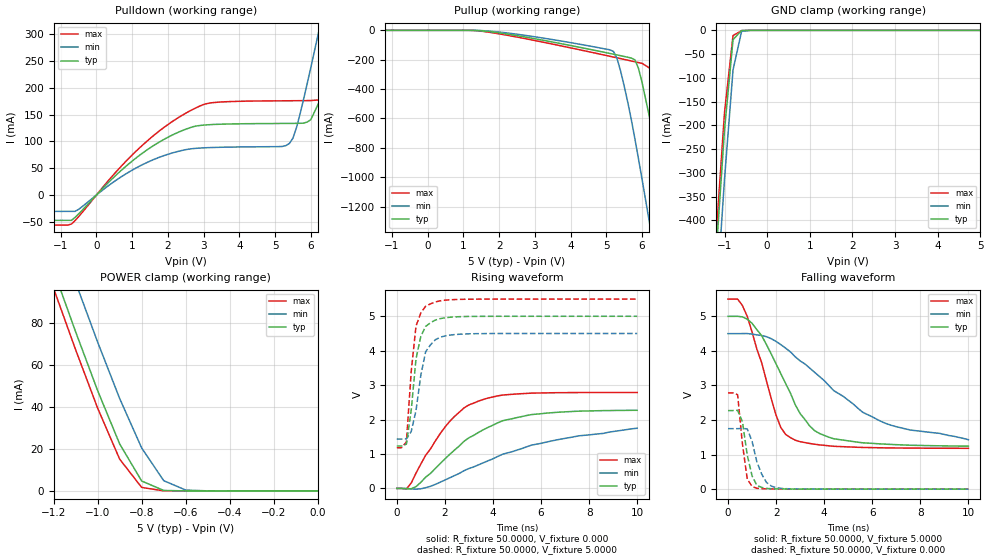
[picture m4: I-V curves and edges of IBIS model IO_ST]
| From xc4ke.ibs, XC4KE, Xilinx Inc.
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|   Model IO_ST
[Model]   IO_ST
Model_type   I/O
Polarity   Non-Inverting
Enable   Active-Low
Vinh  = 2.0V
Vinl  = 0.8V
Vmeas =   2.5000V
Cref =  50.0000pF
Rref =   1.0000M
Vref =  0.000V
C_comp   8.00pF   6.00pF   10.00pF
[Temperature Range]   27.0000   100.0000   0.000
[Voltage Range]   5.0000V   4.5000V   5.5000V
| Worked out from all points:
|   slope of the pulldown table from 0 to 0.75 V, typ, clamps not added: 15.2 ohm
|   GND clamp passes 1 mA (typ) near -0.61 V on its own axis
|   POWER clamp passes 1 mA (typ) near -0.72 V on its own axis
|   rising waveform, R_fixture 50.0000, V_fixture 0.000: 20-80 % time 2.5ns typ, 4.24ns min, 1.74ns max; typ from 0 V to 2.27 V
|   rising waveform, R_fixture 50.0000, V_fixture 5.0000: 20-80 % time 405ps typ, 446ps min, 320ps max; typ from 1.23 V to 5 V
|   falling waveform, R_fixture 50.0000, V_fixture 5.0000: 20-80 % time 1.67ns typ, 3.41ns min, 1.09ns max; typ from 5 V to 1.24 V
|   falling waveform, R_fixture 50.0000, V_fixture 0.000: 20-80 % time 350ps typ, 478ps min, 278ps max; typ from 2.27 V to 0 V
[Pulldown]
| voltage   I(typ)   I(min)   I(max)
-5V       -47.22mA   -30.5mA    -56mA
-700mV    -47.22mA   -30.5mA    -54.14mA
1V        63.37mA    46.41mA    74.73mA
2.5V      122.8mA    84.67mA    152.7mA
5.3V      133.6mA    92.17mA    175.9mA
5.6V      133.8mA    126.2mA    176mA
6V        140.7mA    238mA      176.3mA
6.4V      196.9mA    359.3mA    178.3mA
6.8V      314.8mA    483mA      199.9mA
7.2V      438.1mA    607.8mA    286.2mA
7.6V      562.9mA    733.1mA    407.7mA
10V       1.321A     1.49A      1.163A
[Pullup]
| voltage   I(typ)   I(min)   I(max)
-5V       200pA      348.8pA    219.9pA
1.3V      -437uA     -213.6uA   -1.434mA
5.1V      -157.5mA   -132.9mA   -176.7mA
5.3V      -167.7mA   -191.5mA   -187.3mA
5.4V      -172.8mA   -277.5mA   -192.7mA
5.8V      -201mA     -739.2mA   -214.2mA
6V        -354.6mA   -1.014A    -225.1mA
6.4V      -808.8mA   -1.583A    -285.1mA
6.8V      -1.343A    -2.162A    -713.3mA
7.2V      -1.919A    -2.746A    -1.192A
7.6V      -2.503A    -3.332A    -1.744A
10V       -6.043A    -6.873A    -5.271A
[GND_clamp]
| voltage   I(typ)   I(min)   I(max)
-5V       -6.041A    -6.132A    -6.009A
-1.2V     -475.4mA   -581.5mA   -437mA
-1V       -209.6mA   -313.5mA   -172.9mA
-800mV    -19.58mA   -83.01mA   -10.94mA
-600mV    -371.5uA   -2.252mA   -681.5uA
-400mV    -2.131uA   -13.41uA   -2.859uA
5V        208pA      25.02uA    188.3pA
[POWER_clamp]
| voltage   I(typ)   I(min)   I(max)
-5V       1.297A     1.316A     1.29A
-1.2V     105mA      128.5mA    96.44mA
-1.1V     75.81mA    99.25mA    67.26mA
-1V       47.76mA    70.87mA    39.43mA
-900mV    22.39mA    43.99mA    15.14mA
-800mV    4.715mA    20.43mA    1.664mA
-700mV    224.2uA    4.878mA    49.53uA
-600mV    6.639uA    413.1uA    1.44uA
-500mV    218.8nA    25.05uA    69.52nA
0V        208pA      392.6pA    227.9pA
[Ramp]
| variable   typ   min   max
dV/dt_r   1.3614/2.5013n   1.0008/3.8702n   1.6716/1.6918n
dV/dt_f   2.2536/1.6678n   1.7700/3.1867n   2.5908/1.0296n
R_load = 50.0000
[Rising Waveform]
R_fixture = 50.0000
V_fixture = 0.000
| time   V(typ)   V(min)   V(max)
0s        0V         0V         0V
400ps     -10.76mV   -1.509mV   -15.19mV
800ps     51.43mV    -22.24mV   445.1mV
1.2ns     325.7mV    19.83mV    961.4mV
2.2ns     986.6mV    307mV      1.946V
2.8ns     1.369V     515mV      2.34V
3.4ns     1.627V     685.1mV    2.537V
4.4ns     1.965V     992.6mV    2.712V
5.6ns     2.144V     1.256V     2.767V
10ns      2.269V     1.748V     2.786V
[Rising Waveform]
R_fixture = 50.0000
V_fixture = 5.0000
V_fixture_min = 4.5000
V_fixture_max = 5.5000
| time   V(typ)   V(min)   V(max)
0s        1.231V     1.434V     1.181V
200ps     1.23V      1.434V     1.181V
400ps     1.286V     1.438V     1.349V
600ps     2.267V     1.649V     3.392V
800ps     3.764V     2.262V     4.715V
1ns       4.416V     3.286V     5.095V
1.2ns     4.705V     3.97V      5.291V
1.6ns     4.889V     4.316V     5.417V
2.4ns     4.981V     4.468V     5.486V
10ns      4.999V     4.5V       5.499V
[Falling Waveform]
R_fixture = 50.0000
V_fixture = 5.0000
V_fixture_min = 4.5000
V_fixture_max = 5.5000
| time   V(typ)   V(min)   V(max)
0s        5V         4.5V       5.5V
600ps     4.984V     4.501V     5.312V
1.4ns     4.441V     4.446V     3.659V
2ns       3.624V     4.274V     2.138V
2.2ns     3.337V     4.18V      1.778V
2.6ns     2.773V     3.97V      1.49V
3.4ns     1.827V     3.503V     1.322V
4.4ns     1.458V     2.85V      1.24V
6.6ns     1.3V       1.893V     1.194V
10ns      1.244V     1.43V      1.182V
[Falling Waveform]
R_fixture = 50.0000
V_fixture = 0.000
| time   V(typ)   V(min)   V(max)
0s        2.274V     1.75V      2.786V
400ps     2.282V     1.75V      2.732V
600ps     1.951V     1.759V     1.308V
800ps     987.3mV    1.743V     296.4mV
1ns       387.6mV    1.388V     79.23mV
1.2ns     110.7mV    789.3mV    24.63mV
1.4ns     51.35mV    435.7mV    16.2mV
1.6ns     22.4mV     195mV      8.989mV
2ns       8.353mV    43.99mV    4.854mV
10ns      193.6uV    339.8uV    -100.8uV
